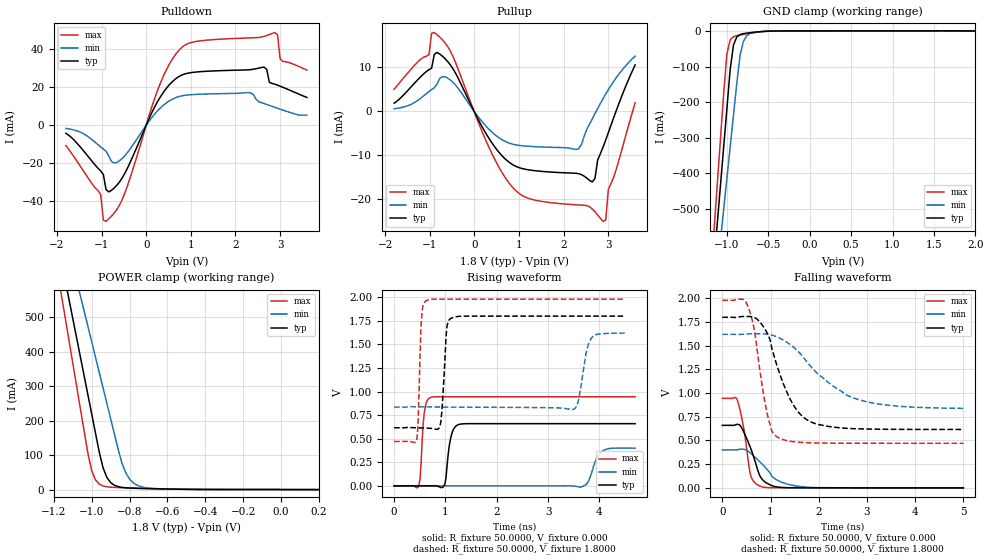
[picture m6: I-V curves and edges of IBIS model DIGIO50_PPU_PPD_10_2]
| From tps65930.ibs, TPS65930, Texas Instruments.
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|   Model DIGIO50_PPU_PPD_10_2
[Model]   DIGIO50_PPU_PPD_10_2
Model_type   I/O
Polarity   Non-Inverting
Enable   Active-Low
Vinl =   0.6900V
Vinh =   1.0500V
Vmeas =   0.9000V
Cref =  30.0000pF
Rref = 100.0000M
Vref =  0.000V
|C_comp   1.4494pF   1.4784pF   1.3595pF
C_comp   30fF   30fF   30fF
[Temperature Range]   25.0000   0.1250k   -40.0000
[Pullup Reference]   1.8000V   1.6200V   1.9800V
[Pulldown Reference]   0.000V   0.000V   0.000V
[POWER Clamp Reference]   1.8000V   1.6200V   1.9800V
[GND Clamp Reference]   0.000V   0.000V   0.000V
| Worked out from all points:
|   slope of the pulldown table from 0 to 0.27 V, typ, clamps not added: 20.8 ohm
|   slope of the pullup table from 0 to 0.27 V, typ, clamps not added: 53.2 ohm
|   GND clamp passes 1 mA (typ) near -0.53 V on its own axis
|   POWER clamp passes 1 mA (typ) near -0.52 V on its own axis
|   rising waveform, R_fixture 50.0000, V_fixture 0.000: 20-80 % time 93.4ps typ, 168ps min, 64.4ps max; typ from 0 V to 0.66 V
|   rising waveform, R_fixture 50.0000, V_fixture 1.8000: 20-80 % time 72ps typ, 148ps min, 51ps max; typ from 0.616 V to 1.8 V
|   falling waveform, R_fixture 50.0000, V_fixture 0.000: 20-80 % time 276ps typ, 458ps min, 169ps max; typ from 0.66 V to 0 V
|   falling waveform, R_fixture 50.0000, V_fixture 1.8000: 20-80 % time 512ps typ, 1.01ns min, 277ps max; typ from 1.8 V to 0.616 V
[Pulldown]
| voltage   I(typ)   I(min)   I(max)
-1.8V     -4.308mA   -1.728mA   -10.75mA
-1.02V    -24.11mA   -11.46mA   -36.55mA
-960mV    -25.97mA   -12.61mA   -49.97mA
-900mV    -33.9mA    -13.68mA   -50.57mA
-600mV    -29.91mA   -18.75mA   -42.1mA
300mV     14.2mA     8.652mA    21.07mA
840mV     26.75mA    15.61mA    41.68mA
2.64V     30.5mA     11.37mA    46.68mA
2.88V     21.54mA    9.385mA    48.69mA
2.94V     21.05mA    8.891mA    47.68mA
3V        20.51mA    8.404mA    34.85mA
3.6V      14.54mA    5.257mA    28.94mA
[Pullup]
| voltage   I(typ)   I(min)   I(max)
-1.8V     1.77mA     483.5uA    4.928mA
-1.02V    9.391mA    4.4mA      12.8mA
-900mV    12.86mA    5.294mA    17.84mA
-540mV    10.48mA    7.032mA    13.62mA
300mV     -5.842mA   -3.922mA   -7.738mA
840mV     -12.14mA   -7.527mA   -17.23mA
2.34V     -14.3mA    -8.546mA   -21.41mA
2.64V     -16.16mA   -1.807mA   -22.34mA
2.88V     -8.283mA   2.786mA    -25.13mA
2.94V     -6.65mA    3.844mA    -24.86mA
3V        -4.947mA   4.856mA    -17.82mA
3.6V      10.48mA    12.48mA    1.856mA
[GND_clamp]
| voltage   I(typ)   I(min)   I(max)
-1.8V     -2.446A    -2.203A    -2.695A
-1.16V    -664.5mA   -773.2mA   -576.6mA
-1.12V    -553mA     -683.7mA   -444.5mA
-1.08V    -441.6mA   -594.2mA   -312.5mA
-1.04V    -330.3mA   -504.7mA   -180.9mA
-1V       -219.1mA   -415.2mA   -65.18mA
-960mV    -108.2mA   -325.7mA   -24.9mA
-920mV    -39.33mA   -236.2mA   -16.07mA
-840mV    -10.22mA   -67.53mA   -11.39mA
-800mV    -7.709mA   -28.93mA   -9.711mA
-720mV    -5.039mA   -7.279mA   -6.548mA
2V        0A         0A         0A
[POWER_clamp]
| voltage   I(typ)   I(min)   I(max)
-1.8V     2.436A     2.212A     2.669A
-1.16V    662mA      785.1mA    563.8mA
-1.12V    551.2mA    695.9mA    432.5mA
-1.06V    385.1mA    562.1mA    235.6mA
-1.02V    274.3mA    472.9mA    104.6mA
-1V       219mA      428.3mA    54.72mA
-960mV    108.4mA    339.2mA    15.79mA
-920mV    35.56mA    250mA      8.195mA
-840mV    6.357mA    76.05mA    5.52mA
-800mV    4.521mA    30.44mA    4.776mA
-760mV    3.691mA    12.55mA    4.076mA
200mV     0A         0A         0A
[Ramp]
| variable   typ   min   max
dV/dt_r   0.3958/0.1489n   0.2403/0.1747n   0.5668/0.5156n
dV/dt_f   0.7102/0.5330n   0.4709/1.0196n   0.9057/0.2904n
R_load = 50.0000
[Rising Waveform]
R_fixture = 50.0000
V_fixture = 0.000
V_fixture_min = 0.000
V_fixture_max = 0.000
| time   V(typ)   V(min)   V(max)
0s        11.15nV    278.2nV    20.93nV
464.6ps   154uV      54.62uV    -16.22mV
585.9ps   194.8uV    44.61uV    766.7mV
707.1ps   530.5uV    37.78uV    935.8mV
989.9ps   19.62mV    26.25uV    944.6mV
1.111ns   526.6mV    22.84uV    944.6mV
1.252ns   649mV      19.53uV    944.6mV
3.636ns   659.6mV    -14.63mV   944.7mV
4.04ns    659.6mV    360.7mV    944.7mV
4.697ns   659.6mV    400.4mV    944.7mV
[Rising Waveform]
R_fixture = 50.0000
V_fixture = 1.8000
V_fixture_min = 1.6200
V_fixture_max = 1.9800
| time   V(typ)   V(min)   V(max)
0s        616.3mV    835.2mV    470.5mV
444.4ps   616mV      839mV      499.3mV
525.3ps   614.6mV    838.3mV    1.703V
626.3ps   612.7mV    837.5mV    1.963V
909.1ps   671.9mV    835.9mV    1.98V
1.03ns    1.692V     835.3mV    1.98V
1.111ns   1.777V     835mV      1.98V
3.485ns   1.8V       809.8mV    1.98V
3.838ns   1.8V       1.563V     1.98V
4.495ns   1.8V       1.62V      1.98V
[Falling Waveform]
R_fixture = 50.0000
V_fixture = 0.000
V_fixture_min = 0.000
V_fixture_max = 0.000
| time   V(typ)   V(min)   V(max)
0s        659.6mV    400.4mV    944.7mV
303ps     669.9mV    401mV      934.4mV
363.6ps   660.8mV    407.3mV    828.9mV
424.2ps   611.2mV    408mV      683.7mV
585.9ps   420.4mV    366.3mV    133.9mV
666.7ps   300.1mV    329.1mV    59.24mV
808.1ps   102.5mV    260.4mV    13.46mV
1.131ns   10.31mV    83.48mV    1.305mV
1.616ns   1.161mV    13.79mV    289.9uV
5ns       815nV      28.54uV    191.8nV
[Falling Waveform]
R_fixture = 50.0000
V_fixture = 1.8000
V_fixture_min = 1.6200
V_fixture_max = 1.9800
| time   V(typ)   V(min)   V(max)
0s        1.8V       1.62V      1.98V
525.3ps   1.808V     1.625V     1.922V
666.7ps   1.798V     1.626V     1.656V
929.3ps   1.633V     1.623V     786.9mV
1.03ns    1.465V     1.612V     596.1mV
1.152ns   1.262V     1.589V     533.3mV
1.515ns   842.1mV    1.468V     485mV
1.919ns   679.3mV    1.234V     474.2mV
2.98ns    621mV      910.4mV    470.6mV
5ns       616.3mV    838.8mV    470.5mV
